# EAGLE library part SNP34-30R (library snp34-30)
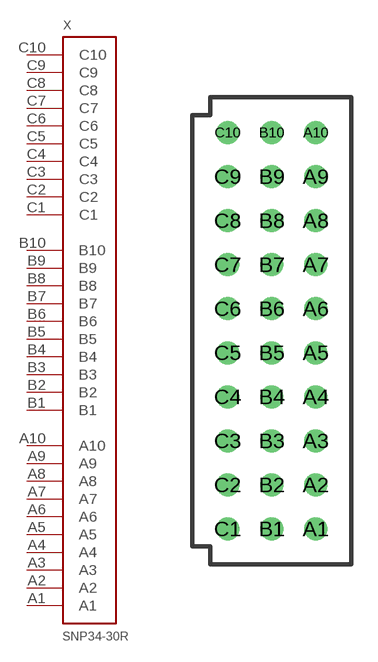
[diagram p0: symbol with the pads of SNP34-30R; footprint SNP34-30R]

Designator prefix X

## SNP34-30R  [SNP34-30R]
A1  A1
A2  A2
A3  A3
A4  A4
A5  A5
A6  A6
A7  A7
A8  A8
A9  A9
A10  A10
B1  B1
B2  B2
B3  B3
B4  B4
B5  B5
B6  B6
B7  B7
B8  B8
B9  B9
B10  B10
C1  C1
C2  C2
C3  C3
C4  C4
C5  C5
C6  C6
C7  C7
C8  C8
C9  C9
C10  C10

## Footprint SNP34-30R (pad centres in mm)
SNP34-30R
drill 0.8: A1 -2,2; A2 -2,4.5; A3 -2,7; A4 -2,9.5; A5 -2,12; A6 -2,14.5; A7 -2,17; A8 -2,19.5; A9 -2,22; A10 -2,24.5; B1 -4.5,2; B2 -4.5,4.5; B3 -4.5,7; B4 -4.5,9.5; B5 -4.5,12; B6 -4.5,14.5; B7 -4.5,17; B8 -4.5,19.5; B9 -4.5,22; B10 -4.5,24.5; C1 -7,2; C2 -7,4.5; C3 -7,7; C4 -7,9.5; C5 -7,12; C6 -7,14.5; C7 -7,17; C8 -7,19.5; C9 -7,22; C10 -7,24.5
